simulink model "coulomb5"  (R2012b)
settings: Solver=ode45  StartTime=0.0  StopTime=10.0  FixedStep=0.001  MaxStep=0.001  RelTol=1e-3
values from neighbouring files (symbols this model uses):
  c = 2200    [coulomb_1.m]    (also in coulomb_10.m = 0.1; coulomb_11.m = 0; coulomb_2.m; coulomb_3.m)
  f = FG    (= 500)    [coulomb_5.m]    (also in dry_friction_1.m; feder_masse_1.m = logspace(e1,e2,5000); feder_masse_11.m = logspace(e1,e2,5000); feder_masse_12.m = logspace(e1,e2,5000))
  Fex_ampl = 800    [coulomb_1.m]    (also in coulomb_2.m; coulomb_3.m; coulomb_4.m; coulomb_5.m)
  fu = 0.02    [coulomb_1.m]    (also in coulomb_2.m; coulomb_3.m; coulomb_4.m; coulomb_5.m = 0.1)
  m = 400    [coulomb_1.m]    (also in coulomb_10.m = 10; coulomb_11.m = 10; coulomb_2.m; coulomb_3.m)
  v0 = 0    [coulomb_1.m]    (also in coulomb_2.m; coulomb_3.m; coulomb_4.m; coulomb_5.m)
  y0 = 0    [coulomb_1.m]    (also in coulomb_2.m; coulomb_3.m; coulomb_4.m; coulomb_5.m)

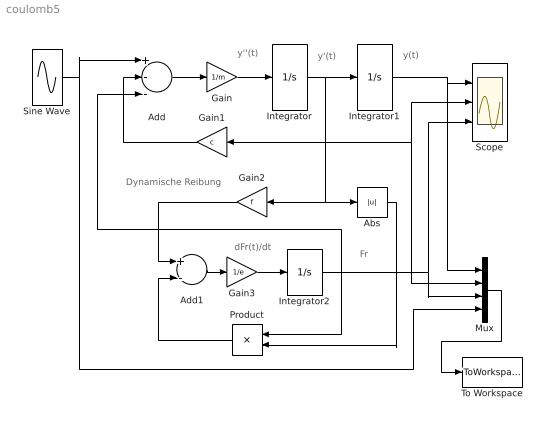
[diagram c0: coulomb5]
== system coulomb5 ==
  note: dFr(t)/dt
  note: Dynamische Reibung
  note: Fr
  note: y(t)
  note: y'(t)
  note: y''(t)
  Abs : Abs
  Add : Sum  Inputs=+--
  Add1 : Sum  Inputs=+-
  Gain : Gain  Gain=1/m
  Gain1 : Gain  Gain=c
  Gain2 : Gain  Gain=f
  Gain3 : Gain  Gain=1/e
  Integrator : Integrator  InitialCondition=v0
  Integrator1 : Integrator  InitialCondition=y0
  Integrator2 : Integrator  ZeroCross=off
  Mux : Mux
  Product : Product
  Scope : Scope  NumInputPorts=3
  Sine Wave : Sin  Amplitude=Fex_ampl  Frequency=fu  SampleTime=0
  To Workspace : ToWorkspace  VariableName=y  SampleTime=-1  SaveFormat=Structure With Time
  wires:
  Add/1 -> Gain/1
  Gain/1 -> Integrator/1
  Gain1/1 -> Add/2
  Gain3/1 -> Integrator2/1
  Add1/1 -> Gain3/1
  Gain2/1 -> Add1/1
  Product/1 -> Add1/2
  Abs/1 -> Product/2
  Integrator1/1 -> Mux/1, Scope/1
  Integrator/1 -> Abs/1, Gain2/1, Mux/2, Scope/2, Gain1/1, Integrator1/1
  Integrator2/1 -> Add/3, Mux/3, Scope/3, Product/1
  Mux/1 -> To Workspace/1
  Sine Wave/1 -> Add/1, Mux/4
